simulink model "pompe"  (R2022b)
settings: Solver=FixedStepAuto  StartTime=0.1  StopTime=5  FixedStep=1e-6  RelTol=1e-3
libraries: simulink x2, dspstat3 x1

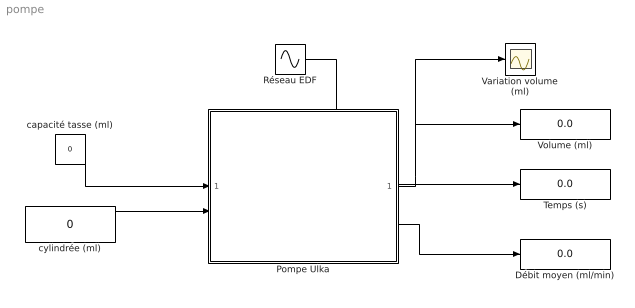
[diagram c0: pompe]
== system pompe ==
  Débit moyen (ml/min) : Display
  Pompe Ulka : Subsystem
  Réseau EDF : Sin  Amplitude=325  Frequency=50*2*pi  SampleTime=0
  Temps (s) : Display
  Variation volume (ml) : Scope
  Volume (ml) : Display
  capacité tasse (ml) : Constant  Value=0
  cylindrée (ml) : Constant  Value=0
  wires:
  Pompe Ulka/1(Out1) -> Variation volume (ml)/1, Volume (ml)/1
  Réseau EDF/1 -> Pompe Ulka/3(u)
  capacité tasse (ml)/1 -> Pompe Ulka/1(In4)
  cylindrée (ml)/1 -> Pompe Ulka/2(In5)
  Pompe Ulka/2(Out2) -> Temps (s)/1
  Pompe Ulka/3(Out3) -> Débit moyen (ml/min)/1

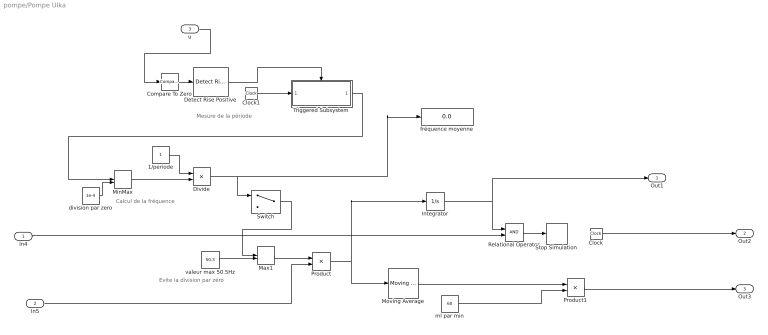
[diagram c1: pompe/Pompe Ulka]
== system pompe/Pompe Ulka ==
  note: Evite la division par zéro
  note: Calcul de la fréquence
  note: Mesure de la période
  In4 : Inport
  In5 : Inport  Port=2
  u : Inport  Port=3
  1/periode : Constant
  Clock : Clock
  Clock1 : Clock
  Compare To Zero : simulink/Logic and Bit Operations/Compare To Zero  relop=<=  OutDataTypeStr=boolean
  Detect Rise Positive : simulink/Logic and Bit Operations/Detect Rise Positive  vinit=0  OutDataTypeStr=boolean
  Divide : Product  Inputs=*/
  Integrator : Integrator
  Max1 : MinMax  Function=max  Inputs=2
  MinMax : MinMax  Function=max  Inputs=2
  Moving Average : dspstat3/Moving Average  Method=Sliding window  ForgettingFactorPort=off  SpecifyWindowLength=on  WindowLength=4  OverlapLength=3  AllowArbitraryInputLength=off  ForgettingFactor=0.9  SimulateUsing=Code generation
  Product : Product
  Product1 : Product
  Relational Operator : RelationalOperator  OutDataTypeStr=boolean  RndMeth=Simplest
  Stop Simulation : Stop
  Switch : Switch  Criteria=u2 > Threshold  Threshold=0.2
  Triggered Subsystem : Subsystem  TreatAsAtomicUnit=on
  division par zero : Constant  Value=1e-4
  fréquence moyenne : Display
  ml par min : Constant  Value=60
  valeur max 50.5Hz : Constant  Value=50.3
  Out1 : Outport
  Out2 : Outport  Port=2
  Out3 : Outport  Port=3
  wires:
  Clock1/1 -> Triggered Subsystem/1(In1)
  Product/1 -> Integrator/1, Moving Average/1
  Detect Rise Positive/1 -> Triggered Subsystem/Trigger
  Compare To Zero/1 -> Detect Rise Positive/1
  ml par min/1 -> Product1/2
  valeur max 50.5Hz/1 -> Max1/2
  1/periode/1 -> Divide/1
  Clock/1 -> Out2/1
  ? -> Switch/3
  Moving Average/1 -> Product1/1
  u/1 -> Compare To Zero/1
  Integrator/1 -> Out1/1, Relational Operator/1
  Relational Operator/1 -> Stop Simulation/1
  Triggered Subsystem/1(Out1) -> MinMax/1
  division par zero/1 -> MinMax/2
  Divide/1 -> Switch/1, fréquence moyenne/1
  MinMax/1 -> Divide/2
  Switch/1 -> Max1/1
  Max1/1 -> Product/1
  In4/1 -> Relational Operator/2
  Product1/1 -> Out3/1
  In5/1 -> Product/2
  ? -> Switch/2

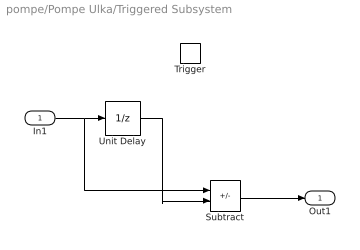
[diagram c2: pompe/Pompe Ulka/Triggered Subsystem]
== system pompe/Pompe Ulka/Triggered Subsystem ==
  In1 : Inport
  Trigger : TriggerPort  VariantControl=(inherit)
  Subtract : Sum  Inputs=+-
  Unit Delay : UnitDelay  SampleTime=-1  HasFrameUpgradeWarning=on
  Out1 : Outport
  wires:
  In1/1 -> Subtract/1, Unit Delay/1
  Unit Delay/1 -> Subtract/2
  Subtract/1 -> Out1/1
